PROGRAM MAIN_CM
VAR CONSTANT
	cInitVibrationAssessment	: ST_CM_VibrationAssessment_InitPars := (	nFFT_Length 		:= cFFTLength, 
																			nWindowLength 		:= cWindowLength,
																			fSampleRate 		:= cSamplerate,
																			nChannels 			:= cChannels,
																			nOrder 				:= cOrder,
																			nMaxBands 			:= cMaxBands,
																			nMaxClasses 		:= cMaxClasses,
																			bMemorize 			:= cMemorize,
																			eWindowType 		:= cWindowType,
																			bTransformToDecibel	:= FALSE,
																			eTraceLevel			:= cTraceLevel);
END_VAR
VAR	
	// VibrationAssessment
	fbVibrationAssessment		: FB_CMA_VibrationAssessment := ( stInitPars := cInitVibrationAssessment, nOwnID := eID_VA, aDestIDs := [eID_Sink] );

	// error monitoring
	fbErrHist					: FB_HRErrHist;

	// Configureation
	bConfigure					: BOOL := TRUE;
	aConfigureClassification	: ARRAY[0..cOrder] OF ARRAY[1..cMaxClasses] OF LREAL;
	aConfigureFrequencyBands	: ARRAY[1..cMaxBands] OF ARRAY[1..2] OF LREAL;
	nClass						: UDINT;
	nBand						: UDINT;
	bReset						: BOOL := FALSE;
END_VAR

IF bConfigure THEN
	(* configure classification *)
	
	FOR nClass := 1 TO cMaxClasses DO
		aConfigureClassification[0][nClass] := cISOClassDef_Vibration[nClass];	// vibration
		aConfigureClassification[1][nClass] := cISOClassDef_Velocity[nClass];	// velocity
		aConfigureClassification[2][nClass] := cISOClassDef_Displ[nClass];		// displacement
	END_FOR
	
	(* configure frequency ranges *)
	
	FOR nBand := 1 TO cMaxBands DO
		aConfigureFrequencyBands[nBand][1] := cfLowerFrequencyLimits[nBand];
		aConfigureFrequencyBands[nBand][2] := cfUpperFrequencyLimits[nBand];	
	END_FOR
	
	(* configure VibrationAssessment *)
	
	fbVibrationAssessment.Configure(	pArg1 := ADR(aConfigureClassification), nArgSize1 := SIZEOF(aConfigureClassification),
										pArg2 := ADR(aConfigureFrequencyBands), nArgSize2 := SIZEOF(aConfigureFrequencyBands));
	IF fbVibrationAssessment.bError THEN
		fbErrHist.AddError(bErr:=TRUE, hrErrCode:=fbVibrationAssessment.hrErrorCode, sErrSource:='MAIN_CM.fbVibrationAssessment.Configure'); // error monitoring
		// ToDo: if error
	ELSE
		bConfigure := FALSE;
	END_IF
END_IF

// Reset data.
IF bReset THEN
	fbVibrationAssessment.ResetData();
	IF fbVibrationAssessment.bError THEN
		fbErrHist.AddError(bErr:=TRUE, hrErrCode:=fbVibrationAssessment.hrErrorCode, sErrSource:='MAIN_CM.fbVibrationAssessment.ResetData'); // error monitoring
		// ToDo: if error
	END_IF
	bReset := FALSE;
END_IF

// Call VibrationAssessment
fbVibrationAssessment.Call();
IF fbVibrationAssessment.bError THEN
	fbErrHist.AddError(bErr:=TRUE, hrErrCode:=fbVibrationAssessment.hrErrorCode, sErrSource:='MAIN_CM.fbVibrationAssessment.Call'); // error monitoring
	// ToDo: if error
END_IF

END_PROGRAM
